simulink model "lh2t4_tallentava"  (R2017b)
settings: Solver=ode45  StartTime=0.0  StopTime=10.0  MaxStep=0.2  RelTol=1e-3  EnableMultiTasking=on
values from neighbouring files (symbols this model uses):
  m0 = 1000    [lh2t4_DOC.m]
  time_to_1 = -1    [lh2t4_DOC.m]
  time_to_2 = 1000    [lh2t4_DOC.m]
libraries: mat24129_lib x3

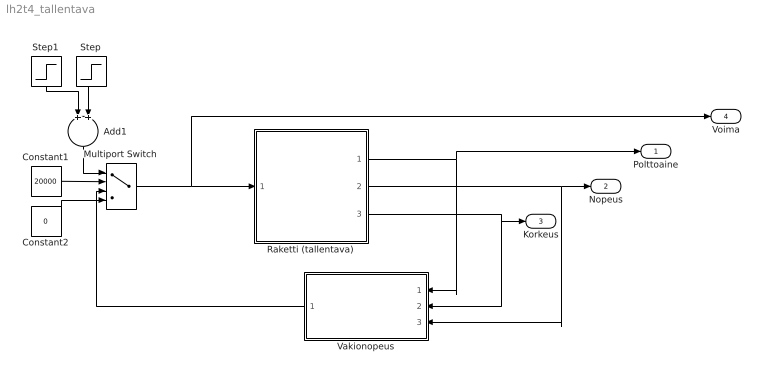
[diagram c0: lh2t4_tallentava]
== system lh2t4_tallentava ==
  Add1 : Sum
  Constant1 : Constant  Value=20000
  Constant2 : Constant  Value=0
  Multiport Switch : MultiPortSwitch  DataPortOrder=Zero-based contiguous  zeroidx=on
  Raketti (tallentava) : Subsystem
  Step : Step  Time=time_to_2  SampleTime=0
  Step1 : Step  Time=time_to_1  SampleTime=0
  Vakionopeus : Subsystem
  Polttoaine : Outport
  Nopeus : Outport  Port=2
  Korkeus : Outport  Port=3
  Voima : Outport  Port=4
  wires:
  Raketti (tallentava)/1(Polttoaine) -> Polttoaine/1, Vakionopeus/1(Polttoaine)
  Vakionopeus/1(Voima) -> Multiport Switch/3
  Constant1/1 -> Multiport Switch/2
  Constant2/1 -> Multiport Switch/4
  Add1/1 -> Multiport Switch/1
  Step1/1 -> Add1/1
  Step/1 -> Add1/2
  Multiport Switch/1 -> Voima/1, Raketti (tallentava)/1(voima)
  Raketti (tallentava)/2(Nopeus) -> Nopeus/1, Vakionopeus/3(Nopeus)
  Raketti (tallentava)/3(Korkeus) -> Korkeus/1, Vakionopeus/2(Korkeus)

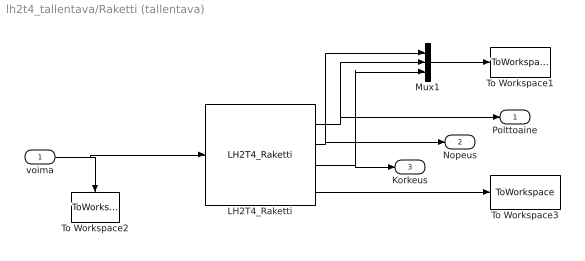
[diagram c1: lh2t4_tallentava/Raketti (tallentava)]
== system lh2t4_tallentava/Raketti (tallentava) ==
  voima : Inport
  LH2T4_Raketti : mat24129_lib/LH2T4_Raketti
  Mux1 : Mux  Inputs=3
  To Workspace1 : ToWorkspace  VariableName=valuesX  SaveFormat=Structure  SampleTime=-1
  To Workspace2 : ToWorkspace  VariableName=valuesU  SaveFormat=Structure  SampleTime=-1
  To Workspace3 : ToWorkspace  VariableName=derivativesX  SaveFormat=Structure  SampleTime=-1
  Polttoaine : Outport
  Nopeus : Outport  Port=2
  Korkeus : Outport  Port=3
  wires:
  voima/1 -> To Workspace2/1, LH2T4_Raketti/1
  Mux1/1 -> To Workspace1/1
  LH2T4_Raketti/1 -> Polttoaine/1, Mux1/2
  LH2T4_Raketti/2 -> Nopeus/1, Mux1/1
  LH2T4_Raketti/3 -> Korkeus/1, Mux1/3
  LH2T4_Raketti/4 -> To Workspace3/1

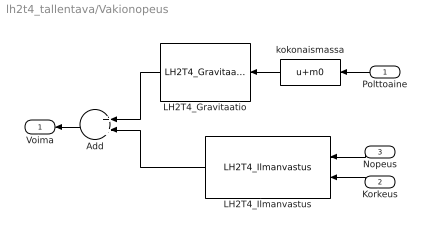
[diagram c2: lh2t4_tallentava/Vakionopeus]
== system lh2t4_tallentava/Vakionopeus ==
  Polttoaine : Inport
  Korkeus : Inport  Port=2
  Nopeus : Inport  Port=3
  Add : Sum
  LH2T4_Gravitaatio : mat24129_lib/LH2T4_Gravitaatio
  LH2T4_Ilmanvastus : mat24129_lib/LH2T4_Ilmanvastus
  kokonaismassa : Fcn  Expr=u+m0
  Voima : Outport
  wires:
  kokonaismassa/1 -> LH2T4_Gravitaatio/1
  LH2T4_Ilmanvastus/1 -> Add/2
  Polttoaine/1 -> kokonaismassa/1
  Nopeus/1 -> LH2T4_Ilmanvastus/1
  Korkeus/1 -> LH2T4_Ilmanvastus/2
  Add/1 -> Voima/1
  LH2T4_Gravitaatio/1 -> Add/1
